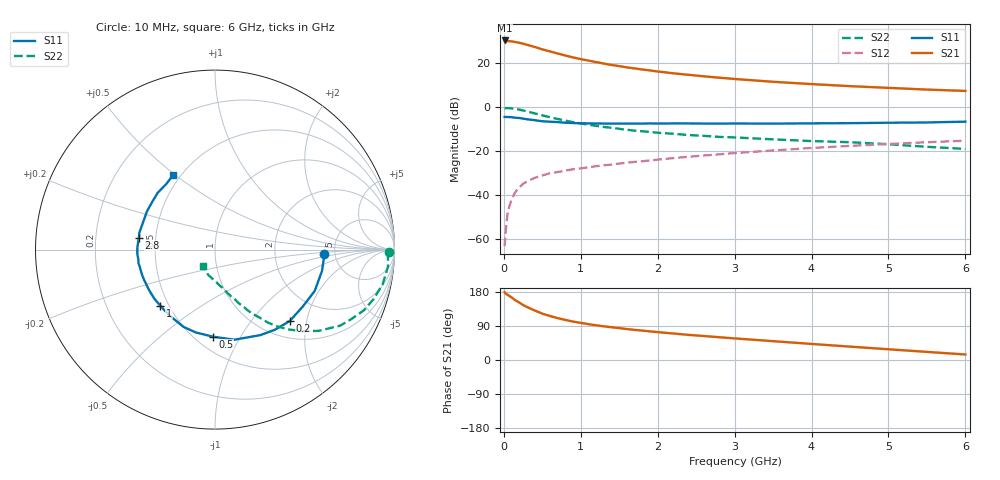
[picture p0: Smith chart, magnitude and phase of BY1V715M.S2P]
! SIEMENS Small Signal Semiconductors
! BFY420
! Si NPN RF SIEGET Grounded Emitter Transistor in MICRO-X
! VCE = 1.75 V  IC = 15 mA
! Common Emitter S-Parameters:  October  1996
# GHz  S  MA  R  50
!  f  S11  S21  S12  S22
! GHz  MAG  ANG  MAG  ANG  MAG  ANG  MAG  ANG
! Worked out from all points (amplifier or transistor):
!   36 points, 10 MHz to 6 GHz, reference 50 ohm
!   highest |S21| = 30.5 dB at 10 MHz (marker M1)
!   |S21| within 3 dB of that: start of sweep to 405.2 MHz
!   unconditionally stable (mu >= 1): 2.144 GHz to end of sweep
!   at 250 MHz: K = 0.25, MSG = 31.9 dB, |S12| = -34.8 dB
!   at 1.4 GHz: K = 0.86, MSG = 22.7 dB, |S12| = -26.0 dB
!   at 6 GHz: K = 1.09, MAG = 9.5 dB, |S12| = -15.1 dB
!   S11 on the Smith chart (normalised r, x): 10 MHz: 4.07, -0.34; 200 MHz: 1.34, -1.59; 500 MHz: 0.61, -0.77; 1 GHz: 0.45, -0.35; 2.8 GHz: 0.40, +0.07; 6 GHz: 0.46, +0.49
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0.01  0.6081 -2.5  33.42 178.9  0.0007 97.5  0.9668 -0.8
0.02  0.6084 -4.8  33.31 176.1  0.0013 97.7  0.9638 -1.9
0.1  0.6014 -22.5  31.87 165.3  0.0081 83.4  0.9542 -11.6
0.15  0.583 -33.0  30.72 157.4  0.0119 76.1  0.9257 -17.3
0.2  0.5761 -43.8  29.67 151.7  0.015 73.8  0.896 -22.2
0.25  0.5572 -53.3  28.19 145.2  0.0183 68.5  0.8527 -27.0
0.3  0.5393 -62.1  26.69 139.8  0.0208 66.0  0.8168 -31.2
0.4  0.5136 -77.8  23.82 130.8  0.025 61.4  0.7338 -38.1
0.5  0.4851 -91.5  20.97 122.3  0.0284 57.8  0.6616 -43.4
0.6  0.4739 -103.1  18.8 116.1  0.0319 55.8  0.5999 -47.7
0.7  0.4648 -112.2  16.9 110.4  0.034 55.0  0.5474 -51.2
0.9  0.4425 -127.7  13.75 101.4  0.0394 53.0  0.4634 -56.1
1  0.4365 -134.4  12.59 97.9  0.0411 52.9  0.433 -58.2
1.1  0.4346 -140.7  11.64 94.6  0.0438 52.9  0.4057 -60.3
1.3  0.4305 -149.5  9.959 88.9  0.0484 52.3  0.3607 -63.1
1.6  0.4302 -161.1  8.156 81.6  0.0553 52.6  0.3106 -67.3
2.2  0.4334 -176.8  5.989 70.0  0.0704 51.4  0.2524 -73.9
2.8  0.4291 171.0  4.753 60.1  0.0858 49.0  0.214 -79.6
3.5  0.429 158.4  3.837 49.7  0.1053 45.2  0.1882 -85.9
4.5  0.4392 142.9  3.052 35.3  0.1337 37.5  0.162 -95.4
5.5  0.4556 126.4  2.552 21.4  0.162 28.6  0.1274 -113.7
6  0.4756 119.6  2.378 14.5  0.1754 23.9  0.114 -127.1
